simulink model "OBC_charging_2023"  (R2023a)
settings: Solver=VariableStepAuto  StartTime=0.0  StopTime=0.1  FixedStep=1e-7  MaxStep=1e-4  RelTol=1e-3
libraries: spsMosfetLib x8, spsSeriesRLCBranchLib x7, spsDiodeLib x4, spsVoltageMeasurementLib x3, spsCurrentMeasurementLib x2, spsACVoltageSourceLib x1, spsMultiWindingTransformerLib x1, spsMultimeterLib x1, simulink x1, spspowerguiLib x1

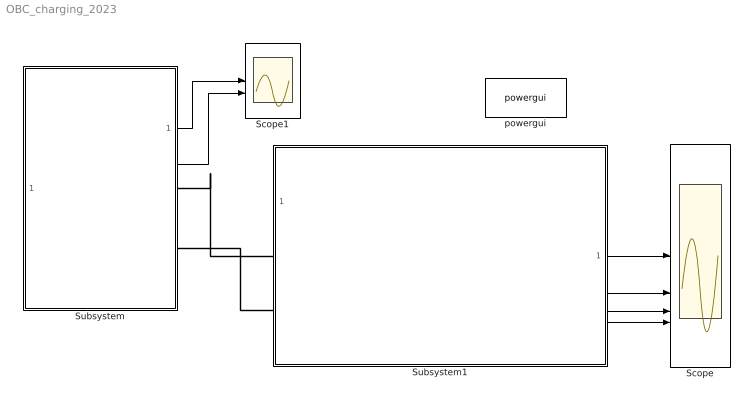
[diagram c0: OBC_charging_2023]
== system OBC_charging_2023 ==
  Scope : Scope  NumInputPorts=4
  Scope1 : Scope  NumInputPorts=2
  Subsystem : Subsystem
  Subsystem1 : Subsystem
  powergui : spspowerguiLib/powergui  Priority=1  SimulationMode=Continuous  SampleTime=50e-6  frequency=60  Iterations=50  frequencyindice=0  Pbase=100e6  ErrMax=1e-4  UnitsV=kV  UnitsW=MW  buscounter=0  FunctionMessages=off  echomessages=off  EnableUseOfTLC=off  CurrentSourceSwitches=off  DisableSnubberDevices=off  DisableRonSwitches=off  DisableVfSwitches=off  DisplayEquations=off  AutomaticDiscreteSolvers=off  SolverType=Tustin/Backward Euler (TBE)  Interpol=off  ExternalGateDelay=off  methode=off  Ts=100  x0status=blocks  SPID=on  SwTol=0  HookPort=off  NonlinearTolerance=1e-4  nMaxIteration=100  ContinueOnMaxIteration=off  RestoreLinks=warning  ResistiveCurrentMeasurement=off  Frange=[0:2:500]  Ylog=off  Xlog=on  ShowGrid=off  save=off  variable=ZData  structure=0  ZoomFFT=off  StartTime=0.0  cycles=1  DisplayStyle=1  fundamental=60  FreqAxis=off  MaxFrequency=1000  frequencyindicesteady=1  RmsSteady=1  display=off
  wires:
  Subsystem1/1(Vbattery) -> Scope/1
  Subsystem1/2(LLC_iLr) -> Scope/2
  Subsystem1/3(Vds_Ids) -> Scope/3
  Subsystem1/4(fsw) -> Scope/4
  Subsystem/1(vac) -> Scope1/1
  Subsystem/2(iac) -> Scope1/2
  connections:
  Subsystem/RConn1 -- Subsystem1/LConn1
  Subsystem1/LConn2 -- Subsystem/RConn2

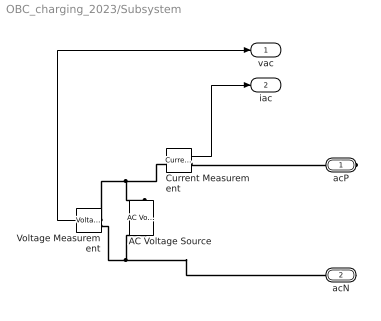
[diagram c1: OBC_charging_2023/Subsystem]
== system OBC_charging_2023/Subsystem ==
  AC Voltage Source : spsACVoltageSourceLib/AC Voltage Source  Amplitude=220*sqrt(2)  Phase=0  Frequency=60  SampleTime=0  Measurements=None  BusType=swing  Pref=10e3  Qref=0  Qmin=-inf  Qmax=+inf
  Current Measurement : spsCurrentMeasurementLib/Current Measurement  PhasorSimulation=off  OutputType=Complex  PSBequivalent=0
  Voltage Measurement : spsVoltageMeasurementLib/Voltage Measurement  PhasorSimulation=off  OutputType=Complex  PSBequivalent=0
  acP : PMIOPort  Side=Right
  acN : PMIOPort  Port=2  Side=Right
  vac : Outport
  iac : Outport  Port=2
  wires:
  Voltage Measurement/1 -> vac/1
  Current Measurement/1 -> iac/1
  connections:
  Voltage Measurement/LConn2 -- acN/RConn1 -- AC Voltage Source/LConn1
  Voltage Measurement/LConn1 -- AC Voltage Source/RConn1 -- Current Measurement/LConn1
  Current Measurement/RConn1 -- acP/RConn1

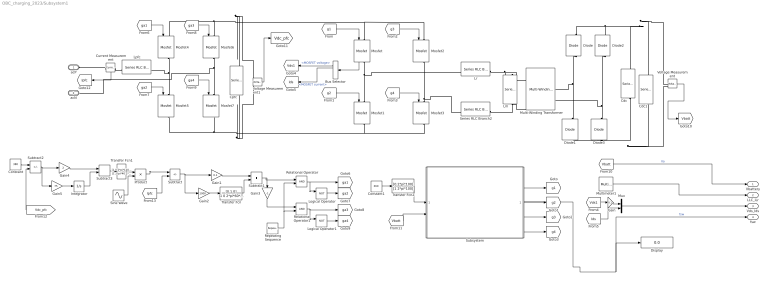
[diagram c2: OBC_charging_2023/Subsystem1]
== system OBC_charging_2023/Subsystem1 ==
  Bus Selector : BusSelector  OutputSignals=MOSFET voltage,MOSFET current
  Cdc : spsSeriesRLCBranchLib/Series RLC Branch  LConnTagsString=__new0  RConnTagsString=__new0  BranchType=C  Resistance=1  Inductance=50.805e-6  SetiL0=off  InitialCurrent=0  Capacitance=1e-3  Setx0=on  InitialVoltage=330  Measurements=Branch voltage
  Cdc1 : spsSeriesRLCBranchLib/Series RLC Branch  LConnTagsString=__new0  RConnTagsString=__new0  BranchType=R  Resistance=20  Inductance=50.805e-6  SetiL0=off  InitialCurrent=0  Capacitance=1e-3  Setx0=on  InitialVoltage=330  Measurements=Branch voltage
  Constant : Constant  Value=380
  Constant1 : Constant  Value=360
  Cpfc : spsSeriesRLCBranchLib/Series RLC Branch  LConnTagsString=__new0  RConnTagsString=__new0  BranchType=C  Resistance=1  Inductance=8.4675e-6  SetiL0=off  InitialCurrent=0  Capacitance=3e-3  Setx0=on  InitialVoltage=400  Measurements=Branch voltage
  Current Measurement : spsCurrentMeasurementLib/Current Measurement  PhasorSimulation=off  OutputType=Complex  PSBequivalent=0
  Diode{,1..3} (4 alike) : spsDiodeLib/Diode  Ron=0.001  Lon=0  Vf=0.8  IC=0  UseSnubber=0  Rs=500  Cs=250e-9  Measurements=on
  Display : Display
  Gain : Gain  Gain=0.1
  Gain1 : Gain  Gain=0.1
  Gain2 : Gain  Gain=1000
  Gain3 : Gain  Gain=-1
  Gain4 : Gain  Gain=2
  Gain5 : Gain  Gain=75
  Integrator : Integrator
  Lm : spsSeriesRLCBranchLib/Series RLC Branch  LConnTagsString=__new0  RConnTagsString=__new0  BranchType=L  Resistance=1  Inductance=50.805e-6  SetiL0=off  InitialCurrent=0  Capacitance=1e-6  Setx0=off  InitialVoltage=0  Measurements=Branch current
  Logical Operator : Logic  Operator=NOT  AllPortsSameDT=off  OutDataTypeStr=boolean
  Logical Operator1 : Logic  Operator=NOT  AllPortsSameDT=off  OutDataTypeStr=boolean
  Lpfc : spsSeriesRLCBranchLib/Series RLC Branch  LConnTagsString=__new0  RConnTagsString=__new0  BranchType=L  Resistance=20  Inductance=5e-3  SetiL0=off  InitialCurrent=0  Capacitance=3e-3  Setx0=on  InitialVoltage=380  Measurements=Branch current
  Lr : spsSeriesRLCBranchLib/Series RLC Branch  LConnTagsString=__new0  RConnTagsString=__new0  BranchType=L  Resistance=1  Inductance=8.4675e-6  SetiL0=off  InitialCurrent=0  Capacitance=1e-6  Setx0=off  InitialVoltage=0  Measurements=Branch current
  Mosfet{,1..7} (8 alike) : spsMosfetLib/Mosfet  Ron=0.1  Lon=0  Rd=0.01  Vfd=0  IC=0  Rs=1e5  Cs=inf  Measurements=on
  Multi-Winding Transformer : spsMultiWindingTransformerLib/Multi-Winding Transformer  LeftWindings=1  RightWindings=1  TappedWindings=no taps  NumberOfTaps=2  SetSaturation=off  Hysteresis=off  DataFile='hysteresis.mat'  Measurements=None  UNITS=pu  NominalPower=[10e3 100e3]  NominalVoltages=[300 300]  WindingResistances=[0.001 0.001]  WindingInductances=[0.001 0.001]  Rm=50  Lm=50  Saturation=[ 0,0 ; 0.0024,1.2 ; 1.0,1.52 ]  SpecifyInitialFlux=off  InitialFlux=0  BreakLoop=off  DiscreteSolver=Trapezoidal iterative  DataType=off  TransfoNumber=1
  Multimeter1 : spsMultimeterLib/Multimeter  L=6  sel=6  yselected={}  Gain=1  OutputType=Complex  PlotAtSimulationStop=off  PhasorSimulation=off
  Mux : Mux  Inputs=2
  Product : Product
  Relational Operator : RelationalOperator  OutDataTypeStr=boolean  RndMeth=Simplest
  Relational Operator1 : RelationalOperator  OutDataTypeStr=boolean  RndMeth=Simplest
  Repeating Sequence : simulink/Sources/Repeating Sequence  rep_seq_t=[0 0.00005]  rep_seq_y=[0 1]
  Series RLC Branch2 : spsSeriesRLCBranchLib/Series RLC Branch  LConnTagsString=__new0  RConnTagsString=__new0  BranchType=C  Resistance=1  Inductance=8.4675e-6  SetiL0=off  InitialCurrent=0  Capacitance=247e-9  Setx0=off  InitialVoltage=0  Measurements=None
  Sine Wave : Sin  Amplitude=-1  Frequency=2*pi*60  SampleTime=0
  Subsystem : Subsystem
  Subtract : Sum  Inputs=+-
  Subtract1 : Sum
  Subtract2 : Sum  Inputs=+-
  Subtract3 : Sum
  Transfer Fcn : TransferFcn  Numerator=[0 1 0]  Denominator=[1 0 2*pi*60*2*pi*60]
  Transfer Fcn1 : TransferFcn  Numerator=[1 0 2*pi*120*2*pi*120]  Denominator=[1 2*pi*40 2*pi*120*2*pi*120]
  Transfer Fcn2 : TransferFcn  Numerator=[0 2*pi*100]  Denominator=[1 2*pi*100]
  Voltage Measurement : spsVoltageMeasurementLib/Voltage Measurement  PhasorSimulation=off  OutputType=Complex  PSBequivalent=0
  Voltage Measurement1 : spsVoltageMeasurementLib/Voltage Measurement  PhasorSimulation=off  OutputType=Complex  PSBequivalent=0
  acP : PMIOPort  Side=Left
  acN : PMIOPort  Port=2  Side=Left
  Vbattery : Outport
  LLC_iLr : Outport  Port=2
  Vds_Ids : Outport  Port=3
  fsw : Outport  Port=4
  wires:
  Subsystem/3(Out3) -> [g2]
  Relational Operator/1 -> [ga1], Logical Operator/1
  [ga1] -> Mosfet4/1
  Subsystem/2(Out2) -> [g1]
  Gain4/1 -> Subtract3/1
  Repeating Sequence/1 -> Relational Operator1/2, Relational Operator/2
  Integrator/1 -> Subtract3/2
  Transfer Fcn2/1 -> Subsystem/1(Vo_ref)
  [g1] -> Mosfet/1
  Subsystem/4(Out4) -> [g3]
  [ga4] -> Mosfet7/1
  Gain1/1 -> Subtract1/1
  Logical Operator1/1 -> [ga4]
  Logical Operator/1 -> [ga2]
  Bus Selector/2 -> [Ids]  "<MOSFET current>"
  Subtract2/1 -> Gain4/1, Gain5/1
  Gain5/1 -> Integrator/1
  [g4] -> Mosfet3/1
  [ga3] -> Mosfet6/1
  Subtract3/1 -> Transfer Fcn1/1
  [Vds1] -> Gain/1
  [g2] -> Mosfet1/1
  Subsystem/5(Out5) -> [g4]
  [Ids] -> Mux/2
  Subtract/1 -> Gain2/1, Gain1/1
  Gain/1 -> Mux/1
  Product/1 -> Subtract/1
  Relational Operator1/1 -> [ga3], Logical Operator1/1
  Transfer Fcn/1 -> Subtract1/2
  Bus Selector/1 -> [Vds1]  "<MOSFET voltage>"
  Constant1/1 -> Transfer Fcn2/1
  Gain2/1 -> Transfer Fcn/1
  Multimeter1/1 -> LLC_iLr/1
  [Vbatt] -> Vbattery/1  "Vo"
  Mosfet/1 -> Bus Selector/1
  [Vbatt] -> Subsystem/2(Vo)
  Subtract1/1 -> Gain3/1, Relational Operator/1
  Mux/1 -> Vds_Ids/1
  Subsystem/1(fsw) -> fsw/1, Display/1  "fsw"
  [ga2] -> Mosfet5/1
  [g3] -> Mosfet2/1
  Gain3/1 -> Relational Operator1/1
  Constant/1 -> Subtract2/1
  Sine Wave/1 -> Product/2
  Transfer Fcn1/1 -> Product/1
  Voltage Measurement/1 -> [Vbatt]
  Voltage Measurement1/1 -> [Vdc_pfc]
  [Vdc_pfc] -> Subtract2/2
  Current Measurement/1 -> [Ipfc]
  [Ipfc] -> Subtract/2
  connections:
  Mosfet3/RConn1 -- Voltage Measurement1/LConn2 -- Cpfc/RConn1 -- Mosfet7/RConn1 -- Mosfet5/RConn1 -- Mosfet1/RConn1
  Mosfet5/LConn1 -- Lpfc/LConn1 -- Mosfet4/RConn1
  Mosfet3/LConn1 -- Mosfet2/RConn1 -- Series RLC Branch2/RConn1
  Mosfet/LConn1 -- Voltage Measurement1/LConn1 -- Cpfc/LConn1 -- Mosfet4/LConn1 -- Mosfet6/LConn1 -- Mosfet2/LConn1
  Lm/RConn1 -- Multi-Winding Transformer/LConn2 -- Series RLC Branch2/LConn1
  Cdc/RConn1 -- Cdc1/RConn1 -- Voltage Measurement/LConn2 -- Diode1/LConn1 -- Diode3/LConn1
  Diode3/RConn1 -- Diode2/LConn1 -- Multi-Winding Transformer/RConn2
  Lr/RConn1 -- Multi-Winding Transformer/LConn1 -- Lm/LConn1
  Diode1/RConn1 -- Diode/LConn1 -- Multi-Winding Transformer/RConn1
  Mosfet6/RConn1 -- acN/RConn1 -- Mosfet7/LConn1
  Diode/RConn1 -- Diode2/RConn1 -- Cdc1/LConn1 -- Voltage Measurement/LConn1 -- Cdc/LConn1
  Mosfet1/LConn1 -- Lr/LConn1 -- Mosfet/RConn1
  Current Measurement/LConn1 -- Lpfc/RConn1
  Current Measurement/RConn1 -- acP/RConn1

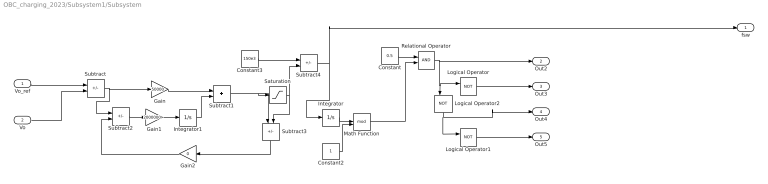
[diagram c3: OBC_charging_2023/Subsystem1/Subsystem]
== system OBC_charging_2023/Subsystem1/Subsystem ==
  Vo_ref : Inport
  Vo : Inport  Port=2
  Constant : Constant  Value=0.5
  Constant2 : Constant
  Constant3 : Constant  Value=150e3
  Gain : Gain  Gain=50000
  Gain1 : Gain  Gain=2000000
  Gain2 : Gain  Gain=0
  Integrator : Integrator
  Integrator1 : Integrator
  Logical Operator : Logic  Operator=NOT  AllPortsSameDT=off  OutDataTypeStr=boolean
  Logical Operator1 : Logic  Operator=NOT  AllPortsSameDT=off  OutDataTypeStr=boolean
  Logical Operator2 : Logic  Operator=NOT  AllPortsSameDT=off  OutDataTypeStr=boolean
  Math Function : Math  Operator=mod
  Relational Operator : RelationalOperator  OutDataTypeStr=boolean  RndMeth=Simplest
  Saturation : Saturate  UpperLimit=60e3  LowerLimit=0
  Subtract{,2..4} (4 alike) : Sum  Inputs=+-
  Subtract1 : Sum
  fsw : Outport
  Out2 : Outport  Port=2
  Out3 : Outport  Port=3
  Out4 : Outport  Port=4
  Out5 : Outport  Port=5
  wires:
  Constant2/1 -> Math Function/2
  Relational Operator/1 -> Out2/1, Logical Operator2/1, Logical Operator/1
  Subtract4/1 -> fsw/1, Integrator/1
  Logical Operator2/1 -> Out4/1, Logical Operator1/1
  Saturation/1 -> Subtract3/2, Subtract4/2
  Subtract1/1 -> Subtract3/1, Saturation/1
  Integrator/1 -> Math Function/1
  Logical Operator1/1 -> Out5/1
  Constant/1 -> Relational Operator/1
  Subtract/1 -> Subtract2/1, Gain/1
  Gain/1 -> Subtract1/1
  Gain2/1 -> Subtract2/2
  Integrator1/1 -> Subtract1/2
  Constant3/1 -> Subtract4/1
  Subtract3/1 -> Gain2/1
  Gain1/1 -> Integrator1/1
  Math Function/1 -> Relational Operator/2
  Subtract2/1 -> Gain1/1
  Vo/1 -> Subtract/2
  Vo_ref/1 -> Subtract/1
  Logical Operator/1 -> Out3/1
